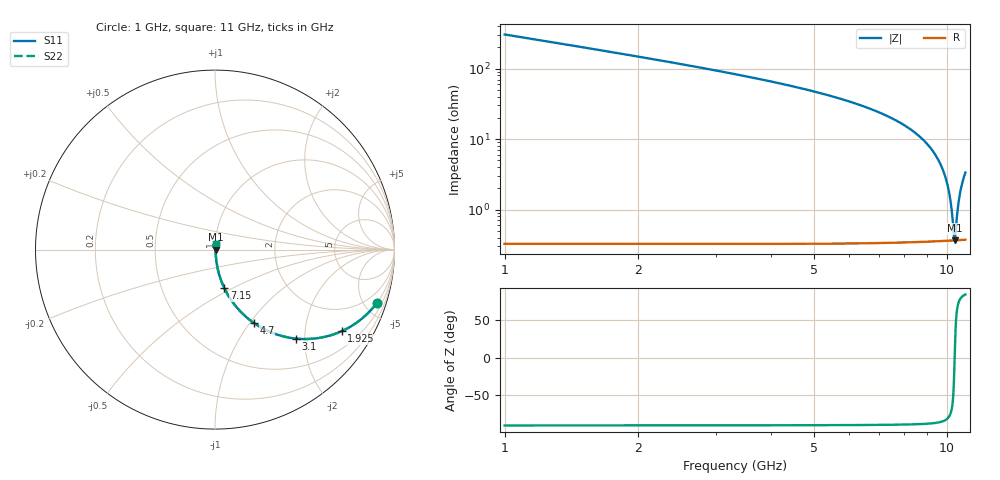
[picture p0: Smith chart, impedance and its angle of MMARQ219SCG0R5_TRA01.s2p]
! MMARQ219SCG0R5_TRA01  S-PARAMETER MODEL  ( General Type )
! Model Generated by TAIYO YUDEN Corporation (http://www.ty-top.com)
! Version 1.0
! TAIYO YUDEN Control No. 160201
! Copyright(c) 2016 TAIYO YUDEN CO.,LTD. All Rights Reserved.
! Product Description (link to TY-COMPAS)
! https://ds.yuden.co.jp/TYCOMPAS/or/detail?pn=MMARQ219SCG0R5BTRA01&u=M
! Products Name : Multilayer Ceramic Capacitors
! Characteristics :
!  Capacitance : 0.5 pF , Rated Voltage : 250V , TCC : CG / C0G
!  Case Size : 2.0 x 1.25 / 0.079 x 0.049 [mm/inch] , Thickness : 0.85 / 0.033 [mm/inch]
!  (Conditions: Temperature = 25 degC , DC Bias Current/Voltage = 0A / 0V)
! External Node Assignments :
!  1  o---| |---o  2
! GND o---------o GND
! Frequency Range : 1000MHz  -  11000MHz  [ 401 STEP ]
# MHz S RI R 50
! Freq[MHz].  S11 Real  S11 Imag  S21 Real  S21 Imag  S12 Real  S12 Imag  S22 Real  S22 Imag
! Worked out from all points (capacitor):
!   401 points, 1 GHz to 11 GHz, reference 50 ohm
!   read as one part in series: C = 516 fF near 1.05 GHz
!   lowest |Z| = 364 mohm at 10.4 GHz (marker M1)
!   series resonance near 10.4 GHz, so ESL is about 450 pH
!   S11 on the Smith chart (normalised r, x): 1 GHz: 1.01, -6.11; 1.925 GHz: 1.01, -3.10; 3.1 GHz: 1.01, -1.81; 4.7 GHz: 1.01, -1.04; 7.15 GHz: 1.01, -0.46; 11 GHz: 1.01, +0.07
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1000  0.903 -0.2954  0.097 0.2954  0.097 0.2954  0.903 -0.2954
1450  0.8127 -0.3893  0.1873 0.3893  0.1873 0.3893  0.8127 -0.3893
1925  0.705 -0.455  0.295 0.455  0.295 0.455  0.705 -0.455
2675  0.5369 -0.4971  0.4631 0.4971  0.4631 0.4971  0.5369 -0.4971
3100  0.4514 -0.4958  0.5486 0.4958  0.5486 0.4958  0.4514 -0.4958
4350  0.2563 -0.4338  0.7437 0.4338  0.7437 0.4338  0.2563 -0.4338
4700  0.2159 -0.4083  0.7841 0.4083  0.7841 0.4083  0.2159 -0.4083
6000  0.1077 -0.3052  0.8923 0.3052  0.8923 0.3052  0.1077 -0.3052
7150  0.0521 -0.2151  0.9479 0.2151  0.9479 0.2151  0.0521 -0.2151
7675  0.0355 -0.1761  0.9645 0.1761  0.9645 0.1761  0.0355 -0.1761
8650  0.0153 -0.108  0.9847 0.108  0.9847 0.108  0.0153 -0.108
9350  0.00747 -0.0627  0.9925 0.0627  0.9925 0.0627  0.00747 -0.0627
9750  0.00501 -0.0381  0.995 0.0381  0.995 0.0381  0.00501 -0.0381
10025  0.00406 -0.0217  0.9959 0.0217  0.9959 0.0217  0.00406 -0.0217
10200  0.00374 -0.0115  0.9963 0.0115  0.9963 0.0115  0.00374 -0.0115
10350  0.00363 -0.00293  0.9964 0.00293  0.9964 0.00293  0.00363 -0.00293
10400  0.00363 -8.64e-05  0.9964 8.64e-05  0.9964 8.64e-05  0.00363 -8.64e-05
10450  0.00364 0.00274  0.9964 -0.00274  0.9964 -0.00274  0.00364 0.00274
10575  0.00375 0.00974  0.9963 -0.00974  0.9963 -0.00974  0.00375 0.00974
10675  0.0039 0.0153  0.9961 -0.0153  0.9961 -0.0153  0.0039 0.0153
10825  0.00424 0.0235  0.9958 -0.0235  0.9958 -0.0235  0.00424 0.0235
11000  0.0048 0.0329  0.9952 -0.0329  0.9952 -0.0329  0.0048 0.0329
